[IBIS ver]   3.2
[File name]   tlk3132.ibs
[File Rev]   1.2
[Date]   May 22, 2009
[Source]   TI
[Copyright]   Copyright 2008 Texas Instruments, Inc.
[Notes]   The following is the IBIS model for the parallel interfaces
   in the TLK3132.  All serial pins should be modeled using
   HSPICE.  All pins associated with the jitter cleaner are
   also not modeled since they are not signal pins
   Rev. 1.1:  Replaced OHSTLTCFVG model with latest ASIC model
   Rev. 1.2:  Added model for REFCLKP(L1)/REFCLKN(K1) pins
|   Component tlk3132
[Component]   TLK3132
[Manufacturer]  TI
[Package]
| variable   typ   min   max
R_pkg   0   0   0
L_pkg   0   0   0
C_pkg   0   0   0
[Pin]   signal_name   model_name   R_pin   L_pin   C_pin
   A1   DGND   GND
   A2   RXD_0   OHSTLTCDVG
   A3   VDDQ   POWER
   A4   RXD_1   OHSTLTCDVG
   A5   RXC_4   OHSTLTCDVG
   A6   RXCLK_0   OHSTLTCDVG
   A7   VDDQ   POWER
   A8   TXD_13   IHSTLTCDVG
   A9   DGND   GND
| A10   RES4   Not modeled
  A11   VREF2   POWER
  A12   TXD_11   IHSTLTCDVG
  A13   TXD_10   IHSTLTCDVG
  A14   TXD_8   IHSTLTCDVG
   B1   RXD_7   OHSTLTCDVG
   B2   RXD_3   OHSTLTCDVG
   B3   DGND   GND
   B4   DGND   GND
   B5   RXCLK_1   OHSTLTCDVG
   B6   VDDQ   POWER
   B7   DGND   GND
   B8   TXD_15   IHSTLTCDVG
   B9   TXC_5   IHSTLTCDVG
  B10   TXD_12   IHSTLTCDVG
  B11   VDDQ   POWER
  B12   TXD_9   IHSTLTCDVG
  B13   VDDQ   POWER
  B14   TXD_7   IHSTLTCDVG
   C1   RXD_9   OHSTLTCDVG
   C2   RXD_4   OHSTLTCDVG
   C3   RXD_6   OHSTLTCDVG
   C4   RXC_5   OHSTLTCDVG
|  C5   RES1   Not modeled
   C6   RXC_1   OHSTLTCDVG
   C7   RXD_2   OHSTLTCDVG
   C8   VPP   POWER
   C9   TXD_14   IHSTLTCDVG
  C10   DGND   GND
  C11   TXD_3   IHSTLTCDVG
  C12   TXD_0   IHSTLTCDVG
  C13   DGND   GND
  C14   TXC_0   IHSTLTCDVG
   D1   VDDQ   POWER
   D2   RXD_8   OHSTLTCDVG
   D3   RXD_11   OHSTLTCDVG
   D4   RXD_13   OHSTLTCDVG
   D5   DGND   GND
   D6   RXD_5   OHSTLTCDVG
   D7   RXC_0   OHSTLTCDVG
   D8   VPP   POWER
   D9   TXC_4   IHSTLTCDVG
  D10   TXCLK_1   IHSTLTCDVG
  D11   TXD_6   IHSTLTCDVG
  D12   TXD_1   IHSTLTCDVG
  D13   TXC_1   IHSTLTCDVG
| D14   RES3   Not modeled
   E1   RXD_10   OHSTLTCDVG
   E2   RXD_12   OHSTLTCDVG
   E3   RXD_14   OHSTLTCDVG
   E4   RXD_15   OHSTLTCDVG
   E5   VDDQ   POWER
   E6   DVDD   POWER
   E7   VDDQ   POWER
   E8   DVDD   POWER
   E9   VDDQ   POWER
  E10   VDDQ   POWER
  E11   DGND   GND
  E12   TXD_5   IHSTLTCDVG
  E13   DGND   GND
  E14   VREF1   POWER
   F1   DGND   GND
   F2   SPEED1   IC25TP18
   F3   VDDO   POWER
   F4   DVDD   POWER
   F5   DVDD   POWER
   F6   DGND   GND
   F7   DGND   GND
   F8   DGND   GND
   F9   DGND   GND
  F10   DVDD   POWER
  F11   TXD_4   IHSTLTCDVG
  F12   TXD_2   IHSTLTCDVG
  F13   MDIO   BQ0457T
  F14   VDDQ   POWER
|  G1   TST_OUT   Not modeled
   G2   VSSA_VCO   GND
|  G3   CP_OUT   Not modeled
   G4   VDDA_VCO   POWER
   G5   VDD_PLL   POWER
   G6   DGND   GND
   G7   DGND   GND
   G8   DGND   GND
   G9   DGND   GND
  G10   DVDD   POWER
  G11   VDDQ   POWER
  G12   TXCLK_0   IHSTLTCDVG
  G13   MDC   BQ0457T
  G14   VDDM   POWER
   H1   REFCLKN   iclkrx18g_MODE0
|  H2   VTUNE   Not modeled
   H3   VDD_CML   POWER
   H4   VSSA_CP   GND
   H5   VSS_PLL   GND
   H6   DGND   GND
   H7   DGND   GND
   H8   DGND   GND
   H9   DGND   GND
  H10   GPO3   OC2525ETFZP18
  H11   GPO1   OC2525ETFZP18
  H12   GPO2   OC2525ETFZP18
  H13   VDDO   POWER
  H14   TDO   OC2525ETFZP18
   J1   REFCLKP   iclkrx18g_MODE0
|  J2   VCO_TL_TST   Not modeled
   J3   VSS_CML   GND
   J4   VDDA_CP   POWER
   J5   DGND   GND
   J6   DGND   GND
   J7   DGND   GND
   J8   DGND   GND
   J9   DGND   GND
  J10   DGND   GND
  J11   PRTAD0   IC25TP18
  J12   TCK   IC25TP18
  J13   SLOOP   IC25TP18
  J14   SPEED0   IC25TP18
   K1   DGND   GND
   K2   REFCLK   IC25TP18
   K3   CODE   IC25TP18
   K4   VDDO   POWER
   K5   DVDD   POWER
   K6   AVDD   POWER
   K7   VDDR   POWER
   K8   AVDD   POWER
   K9   AVDD   POWER
  K10   DVDD   POWER
  K11   AGND   GND
  K12   VDDO   POWER
  K13   TDI   IC25TPUFZP18
  K14   TMS   IC25TPUFZP18
   L1   GPO4   OC2525ETFZP18
   L2   DVDD   POWER
   L3   PRTAD2   BC2525ETFZP18
   L4   AGND   GND
   L5   AGND   GND
   L6   AGND   GND
   L7   VDDR   POWER
   L8   DVDD   POWER
   L9   AGND   GND
  L10   AGND   GND
  L11   AVDD   POWER
  L12   VDDT   POWER
  L13   PRTAD4   IC25TP18
  L14   DGND   GND
   M1   PRBS_EN   IC25TP18
   M2   ENABLE   IC25TP18
   M3   AVDD   POWER
|  M4   TDN0   Not modeled
|  M5   TDP0   Not modeled
   M6   AVDD   POWER
   M7   VDDT   POWER
   M8   AGND   GND
|  M9   RDN0   Not modeled
  M10   VDDT   POWER
| M11   RDP1   Not modeled
  M12   AVDD   POWER
  M13   PLOOP   IC25TP18
  M14   TRST_N   IC25TPUFZP18
   N1   RST_N   IC25TP18
   N2   DVDD   POWER
   N3   PRTAD1   IC25TP18
   N4   AGND   GND
   N5   VDDT   POWER
|  N6   AMUX0   Not modeled
|  N7   TDN1   Not modeled
   N8   VDDT   POWER
|  N9   RDP0   Not modeled
  N10   VDDT   POWER
| N11   RDN1   Not modeled
  N12   AGND   GND
  N13   PRTAD3   IC25TP18
  N14   GPI1   IC25TP18
   P1   DGND   GND
   P2   GPO0   OC2525ETFZP18
   P3   TESTEN   IC25TP18
   P4   VDDD   POWER
   P5   AGND   GND
|  P6   TDP1   Not modeled
   P7   AVDD   POWER
   P8   VDDD   POWER
   P9   AGND   GND
  P10   AVDD   POWER
  P11   VDDD   POWER
  P12   AGND   GND
  P13   VDDD   POWER
  P14   DGND   GND
[Model Selector] BC2525ETFZP18
BC2525ETFZP18_2P5_CO  Cell operated at 2.5(nom)
BC2525ETFZP18_2P5_ID  Cell operated at 2.5(nom)
BC2525ETFZP18_2P5_IN  Cell operated at 2.5(nom)
BC2525ETFZP18_2P5_CM  Cell operated at 2.5(nom)
[Model Selector]   BQ0457T
BQ0457T_12   1.2 volt Vcc
BQ0457T_25A   2.5 volt Vcc
[Model Selector] IC25TP18
IC25TP18_2P5_COM  Cell operated at 2.5(nom)
IC25TP18_2P5_IND  Cell operated at 2.5(nom)
IC25TP18_2P5_IN  Cell operated at 2.5(nom)
IC25TP18_2P5_CM  Cell operated at 2.5(nom)
[Model Selector] IC25TPUFZP18
MODE1_COM5_2P5  Cell operated at 2.5(nom)
MODE4_COM5_2P5  Cell operated at 2.5(nom)
MODE1_IND10_2P5  Cell operated at 2.5(nom)
MODE4_IND10_2P5  Cell operated at 2.5(nom)
MODE1_IND5_2P5  Cell operated at 2.5(nom)
MODE4_IND5_2P5  Cell operated at 2.5(nom)
MODE1_COM10_2P5  Cell operated at 2.5(nom)
MODE4_COM10_2P5  Cell operated at 2.5(nom)
[Model Selector]   IHSTLTCDVG
IHSTLTCDVG0_1P5   Cell operated at VDDS=1.5V(nom) with TRM0=0   TRM1=0
IHSTLTCDVG1_1P5   Cell operated at VDDS=1.5V(nom) with TRM0=VDD TRM1=0
IHSTLTCDVG2_1P5   Cell operated at VDDS=1.5V(nom) with TRM0=0 TRM1=VDD
IHSTLTCDVG3_1P5   Cell operated at VDDS=1.5V(nom) with TRM0=VDD TRM1=VDD
IHSTLTCDVG0_1P8   Cell operated at VDDS=1.8V(nom) with TRM0=0   TRM1=0
IHSTLTCDVG1_1P8   Cell operated at VDDS=1.8V(nom) with TRM0=VDD TRM1=0
IHSTLTCDVG2_1P8   Cell operated at VDDS=1.8V(nom) with TRM0=0 TRM1=VDD
IHSTLTCDVG3_1P8   Cell operated at VDDS=1.8V(nom) with TRM0=VDD TRM1=VDD
[Model Selector] OC2525ETFZP18
OC2525ETFZP18_2P5_CO  Cell operated at 2.5(nom)
OC2525ETFZP18_2P5_ID  Cell operated at 2.5(nom)
OC2525ETFZP18_2P5_IN  Cell operated at 2.5(nom)
OC2525ETFZP18_2P5_CM  Cell operated at 2.5(nom)
[Model Selector] OHSTLTCDVG
SR0SR1_NOTERM_1P5  Cell operated at 1.5(nom)
OSR0NOSR1_NOTERM_1P5  Cell operated at 1.5(nom)
NOSR0SR1_NOTERM_1P5  Cell operated at 1.5(nom)
SR0NOSR1_NOTERM_1P5  Cell operated at 1.5(nom)
SR0SR1_NOTERM_1P8  Cell operated at 1.8(nom)
OSR0NOSR1_NOTERM_1P8  Cell operated at 1.8(nom)
NOSR0SR1_NOTERM_1P8  Cell operated at 1.8(nom)
SR0NOSR1_NOTERM_1P8  Cell operated at 1.8(nom)
| Models and submodels in the file (39): BC2525ETFZP18_2P5_CO (I/O), BC2525ETFZP18_2P5_ID (I/O), BC2525ETFZP18_2P5_IN (I/O), BC2525ETFZP18_2P5_CM (I/O), BQ0457T_12 (I/O), BQ0457T_25A (I/O), IC25TP18_2P5_COM (Input), IC25TP18_2P5_IND (Input), IC25TP18_2P5_IN (Input), IC25TP18_2P5_CM (Input), MODE1_COM5_2P5 (Input), MODE4_COM5_2P5 (Input), MODE1_IND10_2P5 (Input), MODE4_IND10_2P5 (Input), MODE1_IND5_2P5 (Input), MODE4_IND5_2P5 (Input), MODE1_COM10_2P5 (Input), MODE4_COM10_2P5 (Input), iclkrx18g_MODE0 (Input), IHSTLTCDVG0_1P5 (Input), IHSTLTCDVG1_1P5 (Input), IHSTLTCDVG2_1P5 (Input), IHSTLTCDVG3_1P5 (Input), IHSTLTCDVG0_1P8 (Input), IHSTLTCDVG1_1P8 (Input), IHSTLTCDVG2_1P8 (Input), IHSTLTCDVG3_1P8 (Input), OC2525ETFZP18_2P5_CO (3-state), OC2525ETFZP18_2P5_ID (3-state), OC2525ETFZP18_2P5_IN (3-state), OC2525ETFZP18_2P5_CM (3-state), SR0SR1_NOTERM_1P5 (3-state), OSR0NOSR1_NOTERM_1P5 (3-state), NOSR0SR1_NOTERM_1P5 (3-state), SR0NOSR1_NOTERM_1P5 (3-state), SR0SR1_NOTERM_1P8 (3-state), OSR0NOSR1_NOTERM_1P8 (3-state), NOSR0SR1_NOTERM_1P8 (3-state), SR0NOSR1_NOTERM_1P8 (3-state)
